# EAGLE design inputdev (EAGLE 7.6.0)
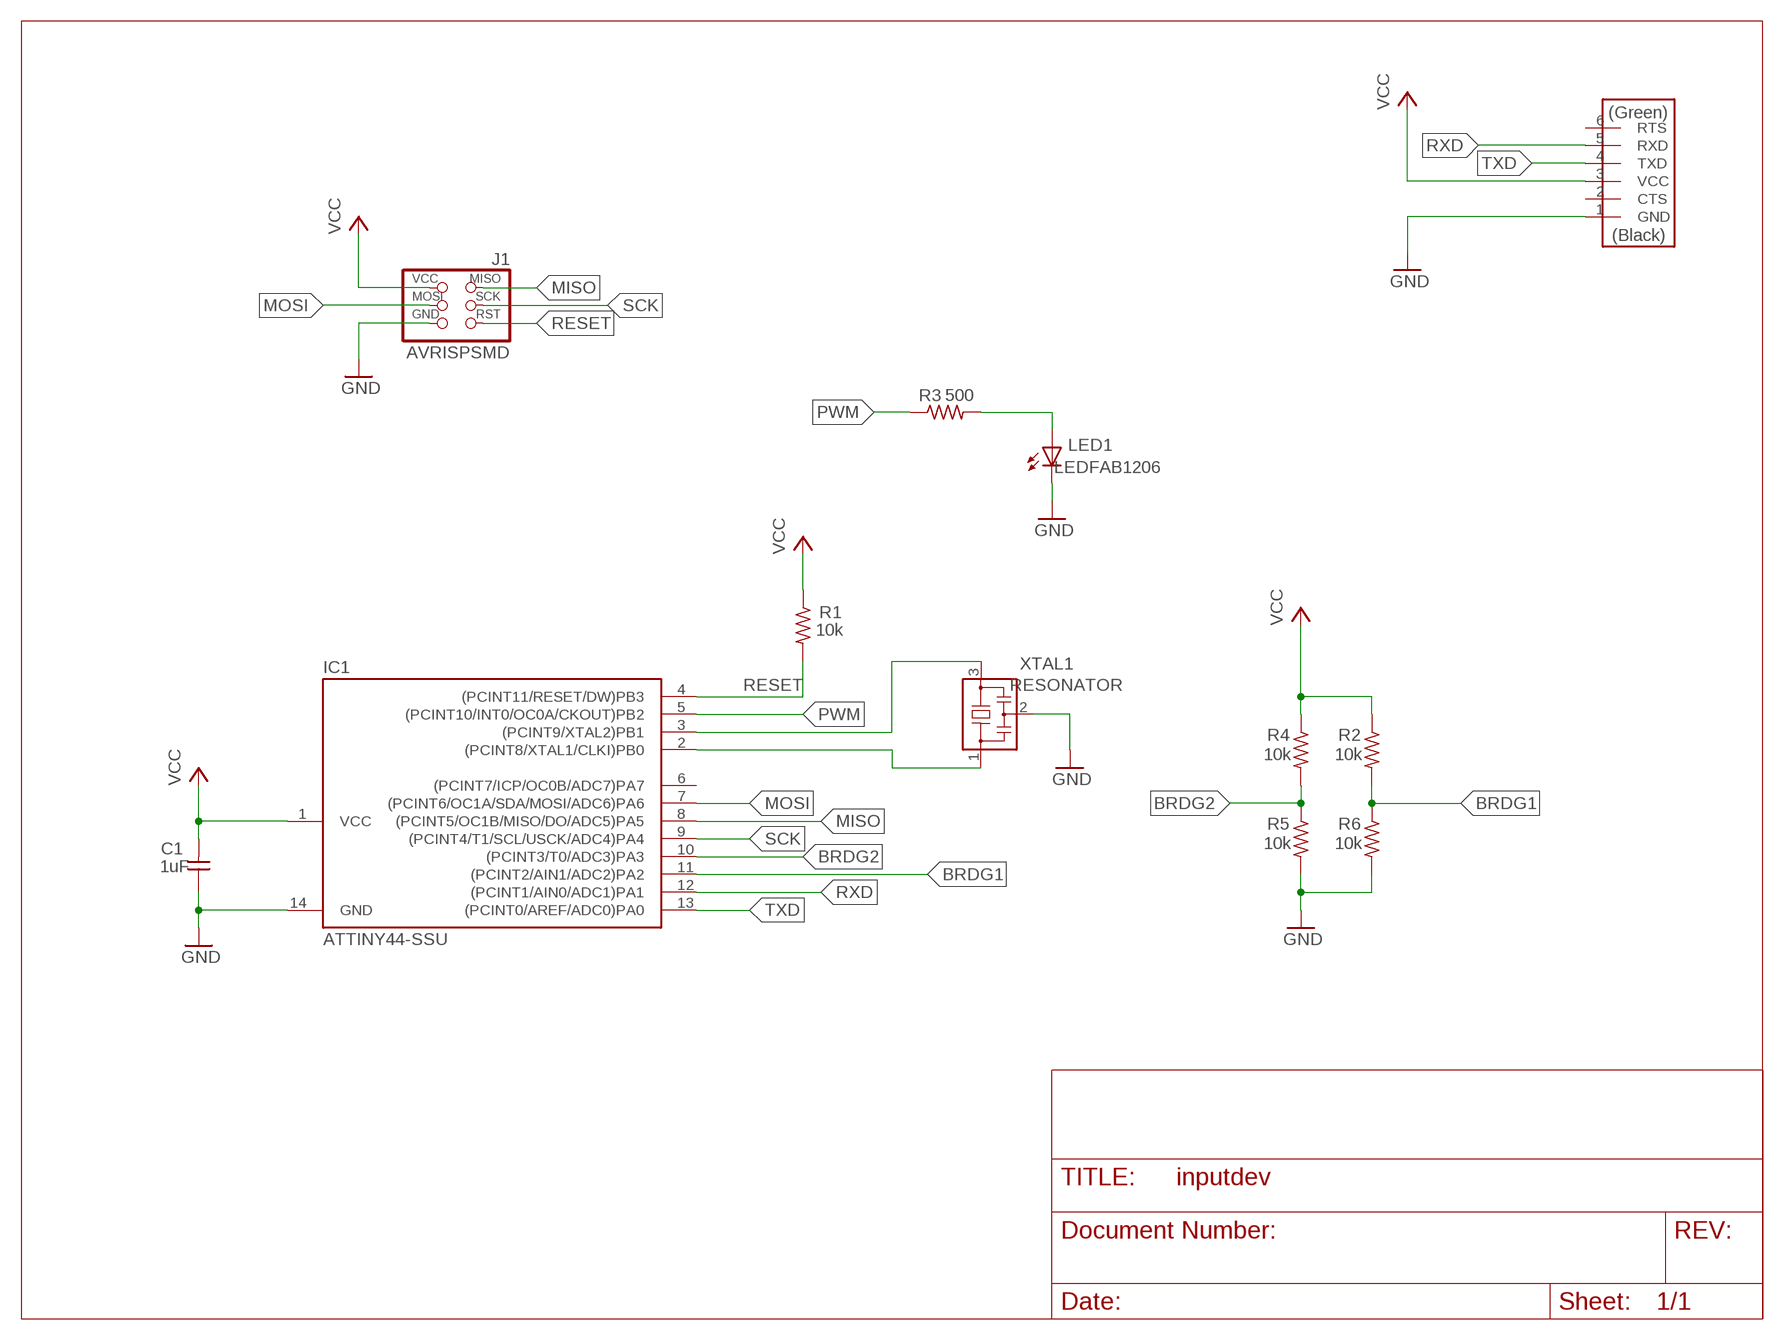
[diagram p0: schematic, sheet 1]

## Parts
C1  1uF  CAP-UNPOLARIZEDFAB  [C1206FAB]
IC1  ATTINY44-SSU  [SOIC14]
J1  AVRISPSMD  [2X03SMD]
J2  FTDI-SMD-HEADER  [1X06SMD]
LED1  LEDFAB1206  [LED1206FAB]
R1  10k  RES-US1206FAB  [R1206FAB]
R2  10k  RES-US1206FAB  [R1206FAB]
R3  500  RES-US1206FAB  [R1206FAB]
R4  10k  RES-US1206FAB  [R1206FAB]
R5  10k  RES-US1206FAB  [R1206FAB]
R6  10k  RES-US1206FAB  [R1206FAB]
XTAL1  RESONATOR  [EFOBM]

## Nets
BRDG1: IC1.11((PCINT2/AIN1/ADC2)PA2) R2.2 R6.1
BRDG2: IC1.10((PCINT3/T0/ADC3)PA3) R4.2 R5.1
GND: C1.1 IC1.14(GND) J1.6(GND) J2.1(GND) LED1.2(C) R5.2 R6.2 XTAL1.2
MISO: IC1.8((PCINT5/OC1B/MISO/DO/ADC5)PA5) J1.1(MISO)
MOSI: IC1.7((PCINT6/OC1A/SDA/MOSI/ADC6)PA6) J1.4(MOSI)
N$1: LED1.1(A) R3.2
N$2: IC1.3((PCINT9/XTAL2)PB1) XTAL1.3
PWM: IC1.5((PCINT10/INT0/OC0A/CKOUT)PB2) R3.1
RESET: IC1.4((PCINT11/RESET/DW)PB3) J1.5(RST) R1.2
RXD: IC1.12((PCINT1/AIN0/ADC1)PA1) J2.5(RXD)
SCK: IC1.9((PCINT4/T1/SCL/USCK/ADC4)PA4) J1.3(SCK)
TXD: IC1.13((PCINT0/AREF/ADC0)PA0) J2.4(TXD)
VCC: C1.2 IC1.1(VCC) J1.2(VCC) J2.3(VCC) R1.1 R2.1 R4.1
XTAL1: IC1.2((PCINT8/XTAL1/CLKI)PB0) XTAL1.1
Unconnected: IC1.6((PCINT7/ICP/OC0B/ADC7)PA7) J2.2(CTS) J2.6(RTS)

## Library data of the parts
C1 = fab:CAP-UNPOLARIZED
IC1 = fab:ATTINY44
J1 = fab:AVRISP
J2 = fab:FTDI-SMD-HEADER
LED1 = fab:LED: LED
R1-R6 = fab:RES-US: Resistor (US Symbol)
XTAL1 = fab:RESONATOR

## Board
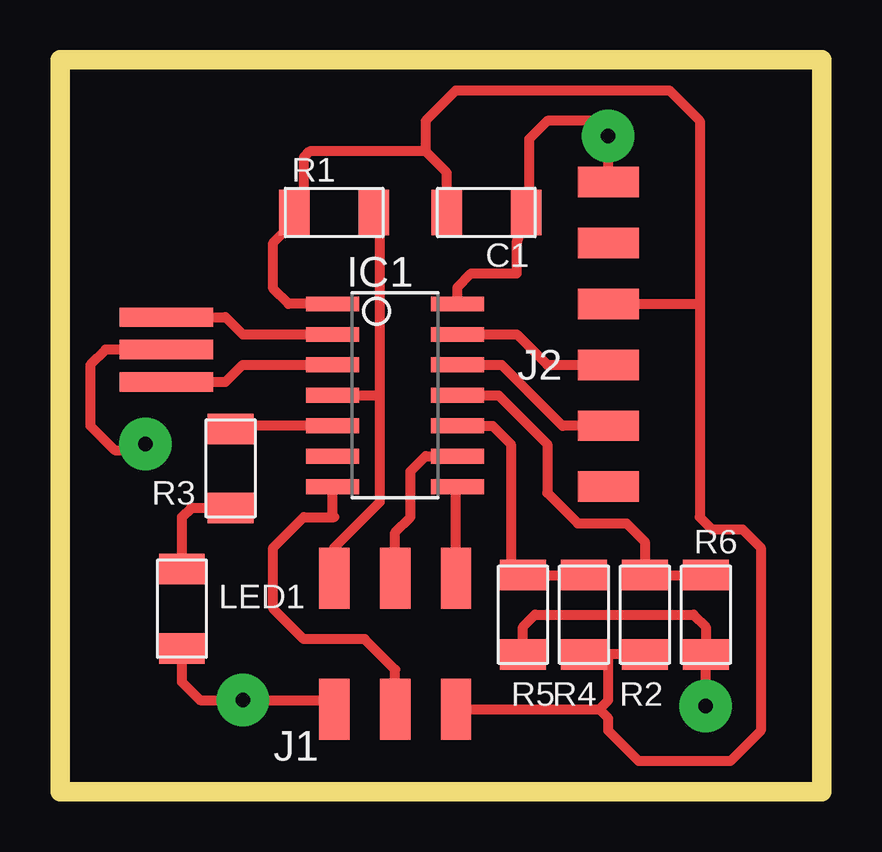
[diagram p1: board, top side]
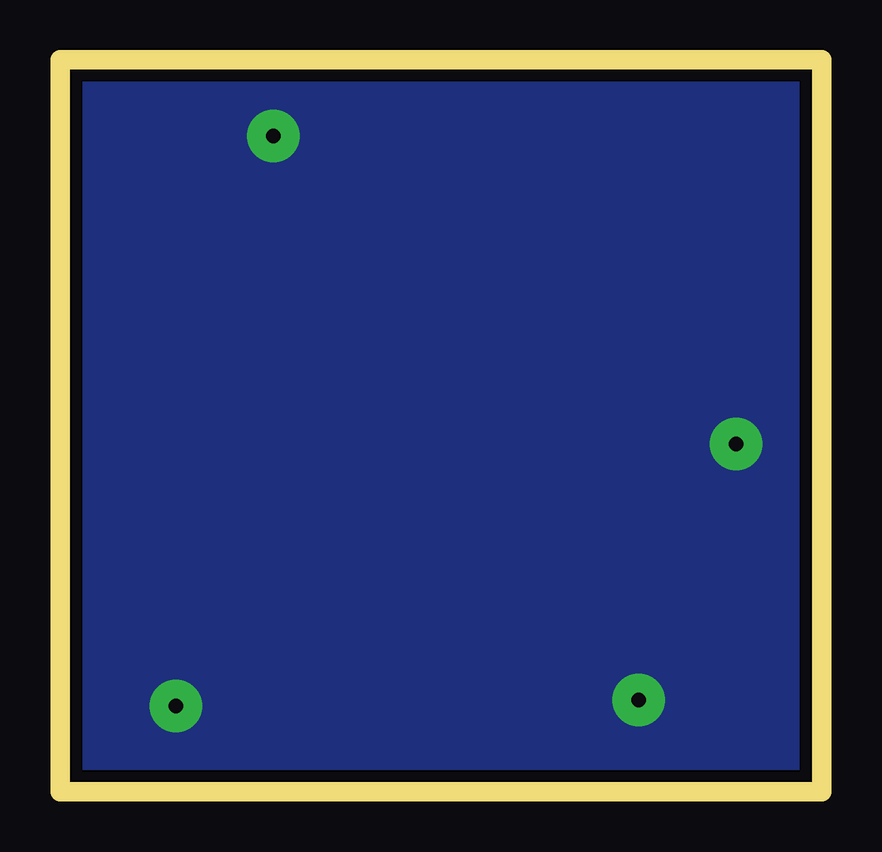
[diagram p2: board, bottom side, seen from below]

Size 31.75 x 30.48 mm. Coordinates in mm from the lower left corner, seen from the top.
Outline: 0,30.48 31.75,30.48 31.75,0 0,0 0,30.48
Copper layers (1*16): Top 0.035mm / dielectric 1.5mm / Bottom 0.035mm
Design rules "default *": minimum track width 12mil, minimum drill 24mil, track to track 17mil, track to pad 16mil, pad to pad 16mil, via to via 16mil, smd to smd 8mil, copper to edge 20mil, drill to drill 8mil, minimum pad ring 10mil, minimum via ring 8mil, stop-mask expansion 4mil, vias tented up to drill 0mil, thermal gap 10mil

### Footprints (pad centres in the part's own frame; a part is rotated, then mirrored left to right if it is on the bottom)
C1206FAB = smd 1.27 x 1.905: 1 -1.651,0; 2 1.651,0
SOIC14 = smd 0.61 x 2.21: 1 -3.81,-2.603; 2 -2.54,-2.603; 3 -1.27,-2.603; 4 0,-2.603; 5 1.27,-2.603; 6 2.54,-2.603; 7 3.81,-2.603; 8 3.81,2.603; 9 2.54,2.603; 10 1.27,2.603; 11 0,2.603; 12 -1.27,2.603; 13 -2.54,2.603; 14 -3.81,2.603
2X03SMD = smd 2.54 x 1.27: 1 -2.54,2.54; 2 2.92,2.54; 3 -2.54,0; 4 2.92,0; 5 -2.54,-2.54; 6 2.92,-2.54
1X06SMD = smd 2.54 x 1.27: 1 0,6.35; 2 0,3.81; 3 0,1.27; 4 0,-1.27; 5 0,-3.81; 6 0,-6.35
LED1206FAB = smd 1.27 x 1.905: 1 -1.651,0; 2 1.651,0
R1206FAB = smd 1.27 x 1.905: 1 -1.651,0; 2 1.651,0
EFOBM = smd 0.8 x 3.9: 1 -1.35,0; 2 0,0; 3 1.35,0

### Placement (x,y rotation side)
C1  17.78,24.13 180 top
IC1  13.97,16.51 270 top
J1  13.97,6.35 270 top
J2  22.86,19.05 0 top
LED1  5.08,7.62 270 top
R1  11.43,24.13 0 top
R2  24.38,7.37 90 top
R3  7.11,13.46 270 top
R4  21.84,7.37 90 top
R5  19.3,7.37 270 top
R6  26.92,7.37 270 top
XTAL1  4.45,18.41 270 top

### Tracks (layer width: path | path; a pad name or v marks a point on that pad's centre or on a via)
BRDG1
  Top 0.406: IC1.11 18.29,16.51 20.32,14.48 20.32,12.45 21.59,11.18 23.62,11.18 24.38,10.41 R2.2 R6.1
BRDG2
  Top 0.406: IC1.10 18.03,15.24 18.8,14.48 18.8,9.52 R5.1 R4.2
GND  (via drill 0.6 pad 2.18)
  Top 0.406: IC1.14 16.57,21.02 17.14,21.59 19.05,21.59 19.05,22.86 C1.1 | 19.05,23.75 C1.1 | C1.1 19.43,24.51 | J2.1 v22.86,27.3 22.86,27.94 20.32,27.94 19.56,27.18 19.56,24.26 C1.1 | R5.2 19.3,6.86 19.81,7.37 26.42,7.37 26.92,6.86 R6.2 v26.92,3.56 | J1.6 11.05,3.81 v7.62,3.81 5.84,3.81 5.08,4.57 LED1.2 | XTAL1.2 1.9,18.41 1.27,17.78 1.27,15.24 2.29,14.22 3.3,14.22 v3.56,14.48
  pour Bottom: 0,30.48 31.75,30.48 31.75,0 0,0
MISO
  Top 0.406: J1.1 16.51,12.64 IC1.8
MOSI
  Top 0.406: J1.4 13.97,5.08 12.7,6.35 10.16,6.35 8.89,7.62 8.89,10.16 10.16,11.43 11.43,11.43 11.37,11.49 IC1.7
N$1
  Top 0.406: R3.2 5.46,11.81 5.08,11.43 LED1.1 5.08,8.89
N$2
  Top 0.406: XTAL1.3 6.9,17.06 7.62,17.78 IC1.3
PWM
  Top 0.406: IC1.5 7.24,15.24 R3.1
RESET
  Top 0.406: J1.5 11.43,10.16 13.33,12.06 13.33,16.51 | IC1.4 13.33,16.51 | 13.33,16.51 13.33,23.49 13.08,23.75 R1.2
RXD
  Top 0.406: IC1.12 18.42,17.78 20.96,15.24 J2.5
SCK
  Top 0.406: J1.3 13.97,10.8 14.61,11.43 14.61,13.34 15.24,13.97 IC1.9
TXD
  Top 0.406: IC1.13 19.05,19.05 20.32,17.78 J2.4
VCC
  Top 0.406: IC1.1 9.52,20.32 8.89,20.95 8.89,22.86 9.78,23.75 R1.1 | C1.2 16.13,25.78 15.24,26.67 | 15.24,26.67 15.24,27.94 16.51,29.21 25.4,29.21 26.67,27.94 26.67,20.32 | R2.1 22.86,5.72 | 22.86,5.72 R4.1 | 9.91,24.26 R1.1 | 15.24,26.67 10.41,26.67 10.16,26.42 10.16,24.51 R1.1 | J1.2 22.48,3.43 | 22.48,3.43 22.86,3.81 22.86,5.72 | J2.3 26.67,20.32 | 26.67,20.32 26.67,11.43 27.18,10.92 28.45,10.92 29.21,10.16 29.21,2.54 27.94,1.27 24.13,1.27 22.86,2.54 22.86,3.05 22.48,3.43
XTAL1
  Top 0.406: XTAL1.1 6.9,19.77 7.62,19.05 IC1.2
